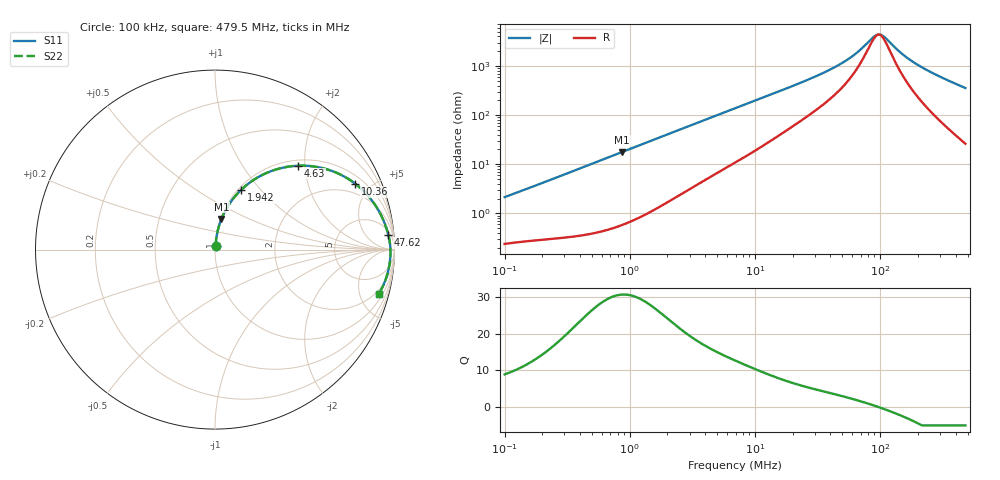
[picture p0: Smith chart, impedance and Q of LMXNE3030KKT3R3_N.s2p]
! LMXNE3030KKT3R3_N  S-PARAMETER MODEL  ( General Type )
! Model Generated by TAIYO YUDEN Corporation (http://www.ty-top.com)
! Version 1.0
! TAIYO YUDEN Control No. 191023NI43SB-FBB
! Copyright(c) 2019 TAIYO YUDEN CO.,LTD. All Rights Reserved.
! Product Description (link to TY-COMPAS)
! https://ds.yuden.co.jp/TYCOMPAS/or/detail?pn=LMXNE3030KKT3R3MN&u=M
! Products Name : Inductors
! Characteristics :
!  Inductance : 3.3 uH , SRF(min) : 64 MHz , DC Resistance(max) : 0.156 Ohm
!  Rated Current : Saturation :1000 mA , Temp Rise : 1030 mA
!  Case Size : 3.0 x 3.0 / 0.118 x 0.118 [mm/inch] , Thickness : 1 / 0.039 [mm/inch]
!  (Conditions: Temperature = 25 degC , DC Bias Current/Voltage = 0A / 0V)
! External Node Assignments :
!  1  o---GGG---o  2
! GND o---------o GND
! Frequency Range : 0.1MHz  -  479.524407MHz  [ 402 STEP ]
# MHz S RI R 50
! Freq[MHz].  S11 Real  S11 Imag  S21 Real  S21 Imag  S12 Real  S12 Imag  S22 Real  S22 Imag
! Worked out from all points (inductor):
!   401 points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, 100 kHz to 479.5 MHz, reference 50 ohm
!   read as one part in series: L = 3.34 uH near 104.3 kHz
!   highest Q = 30.6 at 868.2 kHz (marker M1), where L = 3.25 uH
!   self-resonance near 97.18 MHz
!   S11 on the Smith chart (normalised r, x): 100 kHz: 1.00, +0.04; 1.942 MHz: 1.03, +0.79; 4.63 MHz: 1.12, +1.84; 10.36 MHz: 1.40, +4.04; 47.62 MHz: 8, +21; 479.5 MHz: 1.52, -7.10
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0.1  0.00283 0.0211  0.9972 -0.0211  0.9972 -0.0211  0.00283 0.0211
0.413557  0.0106 0.0836  0.9894 -0.0836  0.9894 -0.0836  0.0106 0.0836
0.868174  0.0357 0.17  0.9643 -0.17  0.9643 -0.17  0.0357 0.17
1.710297  0.117 0.3027  0.883 -0.3027  0.883 -0.3027  0.117 0.3027
1.942154  0.1444 0.3316  0.8556 -0.3316  0.8556 -0.3316  0.1444 0.3316
2.90484  0.2656 0.4171  0.7344 -0.4171  0.7344 -0.4171  0.2656 0.4171
4.629849  0.4622 0.4674  0.5378 -0.4674  0.5378 -0.4674  0.4622 0.4674
7.073061  0.6493 0.439  0.3507 -0.439  0.3507 -0.439  0.6493 0.439
10.35724  0.7825 0.3662  0.2175 -0.3662  0.2175 -0.3662  0.7825 0.3662
16.50777  0.8836 0.261  0.1164 -0.261  0.1164 -0.261  0.8836 0.261
28.6379  0.9413 0.156  0.0587 -0.156  0.0587 -0.156  0.9413 0.156
47.62004  0.9656 0.0829  0.0344 -0.0829  0.0344 -0.0829  0.9656 0.0829
62.72146  0.9726 0.0495  0.0274 -0.0495  0.0274 -0.0495  0.9726 0.0495
86.18795  0.9769 0.0134  0.0231 -0.0134  0.0231 -0.0134  0.9769 0.0134
93.81119  0.9775 0.00394  0.0225 -0.00394  0.0225 -0.00394  0.9775 0.00394
97.87206  0.9777 -0.000797  0.0223 0.000797  0.0223 0.000797  0.9777 -0.000797
104.2953  0.9779 -0.00793  0.0221 0.00793  0.0221 0.00793  0.9779 -0.00793
118.4342  0.9779 -0.0224  0.0221 0.0224  0.0221 0.0224  0.9779 -0.0224
152.7219  0.9761 -0.0526  0.0239 0.0526  0.0239 0.0526  0.9761 -0.0526
201.1535  0.9712 -0.0891  0.0288 0.0891  0.0288 0.0891  0.9712 -0.0891
300.8612  0.955 -0.1534  0.045 0.1534  0.045 0.1534  0.955 -0.1534
479.5244  0.9112 -0.25  0.0888 0.25  0.0888 0.25  0.9112 -0.25
